| TEXAS INSTRUMENTS INCORPORATED
| Standard Linear and Logic Group
| IBIS Model of SN74LVCZ240A
| OCTAL BUFFER/DRIVER WITH 3-STATE OUTPUTS
| This file contains package information for the following:
|  SSOP 20-pin (DB) package as [Component] LVCZ240A_DB
|  TVSOP 20-pin (DGV) package as [Component] LVCZ240A_DGV
|  SOIC 20-pin (DW) package as [Component] LVCZ240A_DW
|  PDIP 20-pin (N) package as [Component] LVCZ240A_N
|  SOP 20-pin (NS) package as [Component] LVCZ240A_NS
|  TSSOP 20-pin (PW) package as [Component] LVCZ240A_PW
| This device can be powered at the following Vccs:
|  3.3 volt Vcc
|  2.7 volt Vcc
| This file provides unique models under the [Model Selector] for each Vcc.
| For operation at a specific Vcc, select the appropriate model after each
| [Model Selector] keyword.
[IBIS Ver]   3.2
[Comment char]  |_char
[File Name]   sn74lvcz240a.ibs
[File Rev]   1.1 | a_die
[Date]   March 23, 2004
[Source]   Data created from TI-SPICE simulations at TI-SLL.
[Notes]   The following is an IBIS list for the LVCZ240A.
   Please contact sllibis@ti.com with questions and
   comments concerning SLL IBIS models.
   - FILE REV HISTORY
   - 1.1 Release IBIS file on 03/23/04
   - Power clamp data deleted as there is no power-clamp diode.
   - Due to the fact that the Device is 5-V Input/Output
   tolarent, the output model has some Non-Monotonic Warnings.
[Disclaimer] Property of Texas Instruments Incorporated.  Unauthorized
   reproduction and/or distribution is strictly prohibited.
   This product is protected under copyright law.
   Created  2004, (C) Copyright  2004, Texas Instruments
   Incorporated, All Rights Reserved
   UNLESS THERE IS A SIGNED, WRITTEN AGREEMENT TO THE
   CONTRARY, TEXAS INSTRUMENTS (TI) IS PROVIDING THE IBIS
   MODELS  AND WITHOUT ANY WARRANTY, EXPRESSED OR
   IMPLIED.  TI assumes no liability for:
   1) the accuracy of the IBIS models provided to your
   company;
   2) the proper functioning of these IBIS Models in your
   design or for any resulting applications; or
   3) infringement of patents, copyrights or intellectual
   property rights resulting from your use of these IBIS
   models.
   TI provides IBIS Models as a service to our customers.
   You and your company shall not distribute, sell or give
   these models to anyone else without prior written
   permission from TI.
   TI reserves the right to make changes to our products or
   to discontinue any semiconductor product or service
   without notice, and advises our customers to obtain the
   latest version of relevant information to verify, before
   placing orders, that the information being relied on is
   current.
   Please be aware that your receipt and use of the IBIS
   information provided shall serve as acceptance of these
   terms and conditions.  If you do not accept these terms,
   you should return or destroy the IBIS models and any
   other accompanying information immediately.
| Component LVCZ240A_DB 20-pin SSOP
[Component]   LVCZ240A_DB
[Manufacturer]   Texas Instruments, Inc.
[Package]
|   typ   min   max
R_pkg   4.000e-02   3.500e-02   5.100e-02
L_pkg   3.495e-09   3.035e-09   4.314e-09
C_pkg   4.200e-13   3.460e-13   5.020e-13
[Pin]   signal_name   model_name   R_pin   L_pin   C_pin
1   N1OE   LVCZ240A_OE   4.900e-02   4.310e-09   5.020e-13
2   1A1   LVCZ240A_IN   4.800e-02   3.903e-09   4.870e-13
3   2Y4   LVCZ240A_OUT   3.500e-02   3.189e-09   3.960e-13
4   1A2   LVCZ240A_IN   3.500e-02   3.036e-09   3.470e-13
5   2Y3   LVCZ240A_OUT   3.500e-02   3.035e-09   3.670e-13
6   1A3   LVCZ240A_IN   3.500e-02   3.035e-09   3.670e-13
7   2Y2   LVCZ240A_OUT   3.500e-02   3.036e-09   3.470e-13
8   1A4   LVCZ240A_IN   3.500e-02   3.189e-09   3.970e-13
9   2Y1   LVCZ240A_OUT   4.700e-02   3.899e-09   4.880e-13
10   GND   GND   5.100e-02   4.314e-09   5.000e-13
11   2A1   LVCZ240A_IN   5.100e-02   4.314e-09   5.000e-13
12   1Y4   LVCZ240A_OUT   4.700e-02   3.899e-09   4.880e-13
13   2A2   LVCZ240A_IN   3.500e-02   3.189e-09   3.970e-13
14   1Y3   LVCZ240A_OUT   3.500e-02   3.036e-09   3.460e-13
15   2A3   LVCZ240A_IN   3.500e-02   3.035e-09   3.670e-13
16   1Y2   LVCZ240A_OUT   3.500e-02   3.035e-09   3.670e-13
17   2A4   LVCZ240A_IN   3.500e-02   3.036e-09   3.460e-13
18   1Y1   LVCZ240A_OUT   3.500e-02   3.189e-09   3.970e-13
19   N2OE   LVCZ240A_IN   4.700e-02   3.899e-09   4.880e-13
20   VCC   POWER   5.100e-02   4.314e-09   5.020e-13
| Component LVCZ240A_DGV 20-pin TVSOP
[Component]   LVCZ240A_DGV
[Manufacturer]   Texas Instruments, Inc.
[Package]
|   typ   min   max
R_pkg   4.400e-02   3.800e-02   4.800e-02
L_pkg   2.561e-09   2.236e-09   2.961e-09
C_pkg   3.420e-13   2.640e-13   4.460e-13
[Pin]   signal_name   model_name   R_pin   L_pin   C_pin
1   N1OE   LVCZ240A_OE   4.400e-02   2.935e-09   4.170e-13
2   1A1   LVCZ240A_IN   4.200e-02   2.869e-09   4.460e-13
3   2Y4   LVCZ240A_OUT   4.300e-02   2.399e-09   3.160e-13
4   1A2   LVCZ240A_IN   4.400e-02   2.236e-09   2.650e-13
5   2Y3   LVCZ240A_OUT   4.600e-02   2.278e-09   2.640e-13
6   1A3   LVCZ240A_IN   4.500e-02   2.274e-09   2.640e-13
7   2Y2   LVCZ240A_OUT   4.400e-02   2.285e-09   2.690e-13
8   1A4   LVCZ240A_IN   4.300e-02   2.452e-09   3.200e-13
9   2Y1   LVCZ240A_OUT   4.400e-02   2.900e-09   4.460e-13
10   GND   GND   4.400e-02   2.961e-09   4.180e-13
11   2A1   LVCZ240A_IN   4.500e-02   2.954e-09   4.180e-13
12   1Y4   LVCZ240A_OUT   4.200e-02   2.847e-09   4.430e-13
13   2A2   LVCZ240A_IN   4.500e-02   2.453e-09   3.190e-13
14   1Y3   LVCZ240A_OUT   4.500e-02   2.297e-09   2.690e-13
15   2A3   LVCZ240A_IN   4.800e-02   2.334e-09   2.680e-13
16   1Y2   LVCZ240A_OUT   4.800e-02   2.335e-09   2.670e-13
17   2A4   LVCZ240A_IN   4.600e-02   2.299e-09   2.680e-13
18   1Y1   LVCZ240A_OUT   4.600e-02   2.457e-09   3.200e-13
19   N2OE   LVCZ240A_IN   4.300e-02   2.848e-09   4.410e-13
20   VCC   POWER   3.800e-02   2.812e-09   4.080e-13
| Component LVCZ240A_DW 20-pin SOIC
[Component]   LVCZ240A_DW
[Manufacturer]   Texas Instruments, Inc.
[Package]
|   typ   min   max
R_pkg   3.800e-02   3.300e-02   4.500e-02
L_pkg   5.012e-09   4.110e-09   6.349e-09
C_pkg   7.170e-13   5.300e-13   8.680e-13
[Pin]   signal_name   model_name   R_pin   L_pin   C_pin
1   N1OE   LVCZ240A_OE   4.200e-02   6.336e-09   8.650e-13
2   1A1   LVCZ240A_IN   4.300e-02   5.542e-09   8.670e-13
3   2Y4   LVCZ240A_OUT   3.400e-02   4.714e-09   7.320e-13
4   1A2   LVCZ240A_IN   3.400e-02   4.377e-09   5.910e-13
5   2Y3   LVCZ240A_OUT   3.600e-02   4.130e-09   5.330e-13
6   1A3   LVCZ240A_IN   3.500e-02   4.111e-09   5.300e-13
7   2Y2   LVCZ240A_OUT   3.400e-02   4.284e-09   5.830e-13
8   1A4   LVCZ240A_IN   3.400e-02   4.634e-09   7.260e-13
9   2Y1   LVCZ240A_OUT   4.000e-02   5.518e-09   8.650e-13
10   GND   GND   4.300e-02   6.349e-09   8.660e-13
11   2A1   LVCZ240A_IN   4.100e-02   6.281e-09   8.610e-13
12   1Y4   LVCZ240A_OUT   4.500e-02   5.561e-09   8.680e-13
13   2A2   LVCZ240A_IN   3.300e-02   4.778e-09   7.420e-13
14   1Y3   LVCZ240A_OUT   3.500e-02   4.414e-09   5.960e-13
15   2A3   LVCZ240A_IN   3.500e-02   4.110e-09   5.330e-13
16   1Y2   LVCZ240A_OUT   3.600e-02   4.130e-09   5.330e-13
17   2A4   LVCZ240A_IN   3.400e-02   4.377e-09   5.910e-13
18   1Y1   LVCZ240A_OUT   3.400e-02   4.714e-09   7.310e-13
19   N2OE   LVCZ240A_IN   4.300e-02   5.569e-09   8.680e-13
20   VCC   POWER   4.200e-02   6.308e-09   8.640e-13
| Component LVCZ240A_N 20-pin PDIP
[Component]   LVCZ240A_N
[Manufacturer]   Texas Instruments, Inc.
[Package]
|   typ   min   max
R_pkg   4.300e-02   3.800e-02   5.000e-02
L_pkg   7.384e-09   4.680e-09   1.032e-08
C_pkg   5.100e-13   2.310e-13   8.210e-13
[Pin]   signal_name   model_name   R_pin   L_pin   C_pin
1   N1OE   LVCZ240A_OE   4.200e-02   9.427e-09   8.100e-13
2   1A1   LVCZ240A_IN   4.600e-02   8.544e-09   4.560e-13
3   2Y4   LVCZ240A_OUT   4.800e-02   7.163e-09   4.350e-13
4   1A2   LVCZ240A_IN   4.000e-02   4.825e-09   2.610e-13
5   2Y3   LVCZ240A_OUT   4.000e-02   5.284e-09   6.480e-13
6   1A3   LVCZ240A_IN   4.000e-02   4.686e-09   2.320e-13
7   2Y2   LVCZ240A_OUT   4.000e-02   6.359e-09   4.890e-13
8   1A4   LVCZ240A_IN   3.800e-02   7.982e-09   4.750e-13
9   2Y1   LVCZ240A_OUT   4.300e-02   9.403e-09   4.750e-13
10   GND   GND   5.000e-02   1.032e-08   8.050e-13
11   2A1   LVCZ240A_IN   5.000e-02   1.028e-08   8.100e-13
12   1Y4   LVCZ240A_OUT   4.300e-02   9.383e-09   4.770e-13
13   2A2   LVCZ240A_IN   3.800e-02   7.978e-09   4.760e-13
14   1Y3   LVCZ240A_OUT   4.000e-02   6.302e-09   4.920e-13
15   2A3   LVCZ240A_IN   4.000e-02   4.680e-09   2.310e-13
16   1Y2   LVCZ240A_OUT   4.000e-02   5.284e-09   6.480e-13
17   2A4   LVCZ240A_IN   4.000e-02   4.822e-09   2.610e-13
18   1Y1   LVCZ240A_OUT   4.700e-02   7.118e-09   4.390e-13
19   N2OE   LVCZ240A_IN   4.600e-02   8.492e-09   4.610e-13
20   VCC   POWER   4.300e-02   9.348e-09   8.210e-13
| Component LVCZ240A_NS 20-pin SOP
[Component]   LVCZ240A_NS
[Manufacturer]   Texas Instruments, Inc.
[Package]
|   typ   min   max
R_pkg   4.400e-02   2.900e-02   5.800e-02
L_pkg   3.666e-09   2.317e-09   5.115e-09
C_pkg   5.480e-13   3.160e-13   7.250e-13
[Pin]   signal_name   model_name   R_pin   L_pin   C_pin
1   N1OE   LVCZ240A_OE   5.800e-02   5.115e-09   7.250e-13
2   1A1   LVCZ240A_IN   5.300e-02   4.591e-09   7.240e-13
3   2Y4   LVCZ240A_OUT   4.900e-02   3.754e-09   5.720e-13
4   1A2   LVCZ240A_IN   2.900e-02   2.549e-09   3.880e-13
5   2Y3   LVCZ240A_OUT   3.100e-02   2.317e-09   3.160e-13
6   1A3   LVCZ240A_IN   3.100e-02   2.317e-09   3.160e-13
7   2Y2   LVCZ240A_OUT   2.900e-02   2.556e-09   3.990e-13
8   1A4   LVCZ240A_IN   4.900e-02   3.754e-09   5.790e-13
9   2Y1   LVCZ240A_OUT   5.300e-02   4.591e-09   7.240e-13
10   GND   GND   5.800e-02   5.115e-09   7.250e-13
11   2A1   LVCZ240A_IN   5.800e-02   5.115e-09   7.250e-13
12   1Y4   LVCZ240A_OUT   5.300e-02   4.591e-09   7.240e-13
13   2A2   LVCZ240A_IN   4.900e-02   3.754e-09   5.790e-13
14   1Y3   LVCZ240A_OUT   2.900e-02   2.557e-09   3.990e-13
15   2A3   LVCZ240A_IN   3.100e-02   2.317e-09   3.160e-13
16   1Y2   LVCZ240A_OUT   3.100e-02   2.317e-09   3.160e-13
17   2A4   LVCZ240A_IN   2.900e-02   2.557e-09   3.990e-13
18   1Y1   LVCZ240A_OUT   4.900e-02   3.754e-09   5.790e-13
19   N2OE   LVCZ240A_IN   5.300e-02   4.591e-09   7.240e-13
20   VCC   POWER   5.800e-02   5.115e-09   7.250e-13
| Component LVCZ240A_PW 20-pin TSSOP
[Component]   LVCZ240A_PW
[Manufacturer]   Texas Instruments, Inc.
[Package]
|   typ   min   max
R_pkg   5.000e-02   4.200e-02   6.000e-02
L_pkg   2.802e-09   2.248e-09   3.553e-09
C_pkg   3.170e-13   2.020e-13   4.430e-13
[Pin]   signal_name   model_name   R_pin   L_pin   C_pin
1   N1OE   LVCZ240A_OE   5.500e-02   3.461e-09   4.400e-13
2   1A1   LVCZ240A_IN   5.500e-02   3.150e-09   4.010e-13
3   2Y4   LVCZ240A_OUT   4.200e-02   2.619e-09   3.020e-13
4   1A2   LVCZ240A_IN   4.500e-02   2.273e-09   2.020e-13
5   2Y3   LVCZ240A_OUT   4.500e-02   2.248e-09   2.240e-13
6   1A3   LVCZ240A_IN   4.500e-02   2.273e-09   2.260e-13
7   2Y2   LVCZ240A_OUT   4.400e-02   2.323e-09   2.050e-13
8   1A4   LVCZ240A_IN   4.600e-02   2.704e-09   3.070e-13
9   2Y1   LVCZ240A_OUT   6.000e-02   3.265e-09   4.110e-13
10   GND   GND   5.700e-02   3.506e-09   4.360e-13
11   2A1   LVCZ240A_IN   5.800e-02   3.553e-09   4.370e-13
12   1Y4   LVCZ240A_OUT   5.800e-02   3.193e-09   4.050e-13
13   2A2   LVCZ240A_IN   4.200e-02   2.704e-09   3.110e-13
14   1Y3   LVCZ240A_OUT   4.600e-02   2.392e-09   2.100e-13
15   2A3   LVCZ240A_IN   4.700e-02   2.334e-09   2.290e-13
16   1Y2   LVCZ240A_OUT   4.700e-02   2.300e-09   2.270e-13
17   2A4   LVCZ240A_IN   4.700e-02   2.349e-09   2.070e-13
18   1Y1   LVCZ240A_OUT   4.500e-02   2.677e-09   3.060e-13
19   N2OE   LVCZ240A_IN   6.000e-02   3.235e-09   4.060e-13
20   VCC   POWER   5.600e-02   3.487e-09   4.430e-13
| Model LVCZ240A_IN
[Model Selector]   LVCZ240A_IN
LVCZ240A_IN_33   3.3 volt Vcc
LVCZ240A_IN_27   2.7 volt Vcc
| Model LVCZ240A_OE
[Model Selector]   LVCZ240A_OE
LVCZ240A_OE_33   3.3 volt Vcc
LVCZ240A_OE_27   2.7 volt Vcc
| Model LVCZ240A_OUT
[Model Selector]   LVCZ240A_OUT
LVCZ240A_OUT_33   3.3 volt Vcc
LVCZ240A_OUT_27   2.7 volt Vcc
| Models and submodels in the file (6): LVCZ240A_IN_33 (Input), LVCZ240A_IN_27 (Input), LVCZ240A_OE_33 (Input), LVCZ240A_OE_27 (Input), LVCZ240A_OUT_33 (3-state), LVCZ240A_OUT_27 (3-state)
